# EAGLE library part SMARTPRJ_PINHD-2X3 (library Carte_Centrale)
PIN HEADER
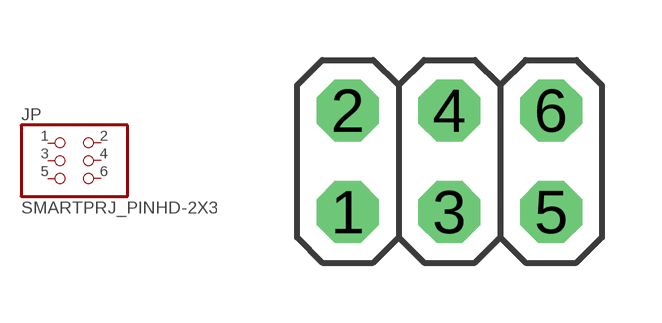
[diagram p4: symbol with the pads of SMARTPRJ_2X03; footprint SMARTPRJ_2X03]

Designator prefix JP

## SMARTPRJ_PINHD-2X3  [SMARTPRJ_2X03]
1  1  pas
2  2  pas
3  3  pas
4  4  pas
5  5  pas
6  6  pas

## Footprint SMARTPRJ_2X03 (pad centres in mm)
PIN HEADER
drill 0.95 pad 1.55 octagon: 1 -2.54,-1.27; 2 -2.54,1.27; 3 0,-1.27; 4 0,1.27; 5 2.54,-1.27; 6 2.54,1.27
